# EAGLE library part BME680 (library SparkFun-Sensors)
Bosch BME680 &ndash; Combined Humidity and Pressure Sensor The BME680 is as combined digital humidity, pressure and temperature sensor based on proven sensing principles. The sensor module is housed in an extremely compact metal-lid LGA package with a footprint of only 3.0×3.0mm² with a height of 0.93mm. Its small dimensions and its low power consumption allow the implementation in battery driven devices such as handsets, GPS modules or watches.
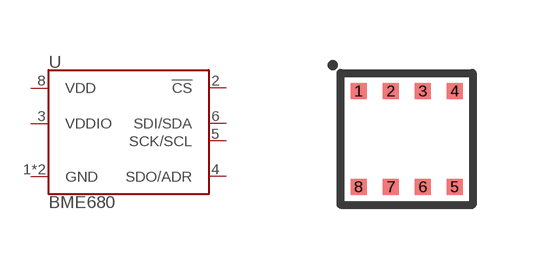
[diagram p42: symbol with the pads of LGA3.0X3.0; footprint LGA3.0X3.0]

Designator prefix U

## BME680BME680  [LGA3.0X3.0]
1  GND
2  !CS
3  VDDIO
4  SDO/ADR
5  SCK/SCL
6  SDI/SDA
7  GND
8  VDD

## Footprint LGA3.0X3.0 (pad centres in mm)
smd 0.4 x 0.4: 1 -1.2,1.2; 2 -0.4,1.2; 3 0.4,1.2; 4 1.2,1.2; 5 1.2,-1.2; 6 0.4,-1.2; 7 -0.4,-1.2; 8 -1.2,-1.2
